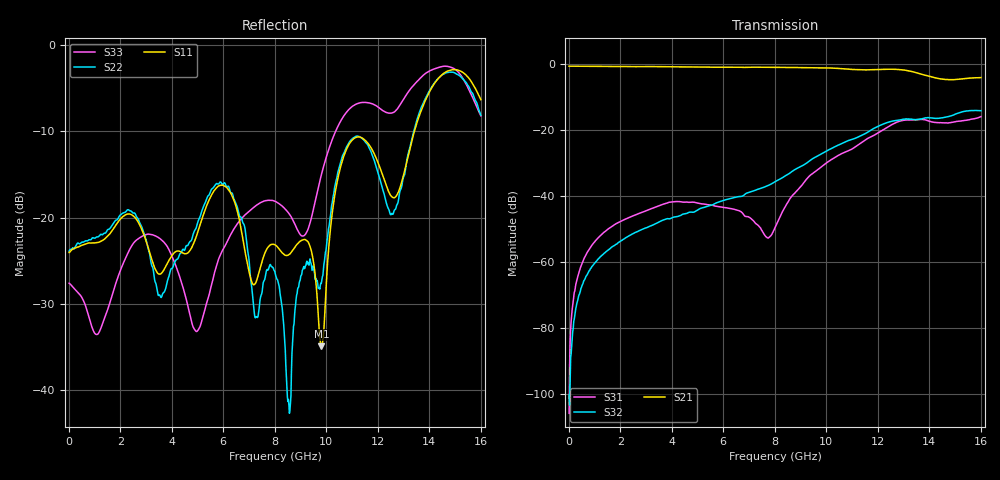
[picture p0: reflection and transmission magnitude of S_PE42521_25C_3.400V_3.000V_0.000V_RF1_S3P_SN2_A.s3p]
! Device ID: PE42521_Char_Units
! Serial: 2
! Insertion: A
! Temp: 25C
! VDD: 3.400
! Control_Hi: 3.000
! Control_Lo: 0.000
! Logic State: RF1
! ThroughPath: 2-1
! Port 1: RFC
! Port 2: RF1
! Port 3: RF2
! V1 = 3.00
! V2 = 0.00
! V3 = 0.00
! IDD: 1.364295e-04
! FILE NAME
! DATE 07-24-2013 19:14:31
! CORRECTED  DATA
#  Hz  S  RI  R  50
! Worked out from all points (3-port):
!   801 points, 10 MHz to 16.01 GHz, reference 50 ohm
!   strongest paths, dB at 10 MHz, 4.01 GHz, 8.01 GHz, 12.01 GHz, 16.01 GHz:
!     S21: -0.6, -0.8, -1.0, -1.6, -4.1
!     S32: -100.1, -46.5, -35.6, -18.8, -14.1
!     S31: -105.7, -41.7, -49.5, -20.9, -15.9
!   lowest |S11| = -34.9 dB at 9.81 GHz (marker M1), VSWR 1.04, Z = 48.5 - j1.02 ohm
!   |S11| at or under -10 dB: start of sweep to 13.43 GHz
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1e7  0.0628 -3.97e-05  0.9287 -0.00284  5.22e-06 2.55e-07
     0.9301 -0.00297  0.064 -0.000303  -3.27e-08 -1.37e-06
     1.71e-06 -4.88e-06  -3.36e-06 -9.25e-06  -0.0417 0.000256
6.5e8  0.0691 -0.0135  0.9117 -0.1498  -8.36e-05 0.00126
       0.9131 -0.1493  0.0721 -0.0132  -0.000164 0.000569
       -8.46e-05 0.00126  -0.000154 0.000567  -0.0306 0.00397
2.09e9  0.0892 0.0477  0.798 -0.4441  0.00125 0.00413
        0.7997 -0.4446  0.0944 0.0484  -9.73e-05 0.00219
        0.00125 0.00413  -0.000107 0.00219  -0.00571 0.0531
4.99e9  0.0701 -0.0402  0.3118 -0.8479  0.00671 0.00416
        0.3142 -0.8475  0.0725 -0.0565  0.000837 0.0061
        0.00673 0.00417  0.000821 0.00606  0.00249 -0.0219
8.01e9  -0.0577 -0.0389  -0.3495 -0.8197  -0.00105 0.00311
        -0.3457 -0.8202  -0.0383 0.0294  0.00327 0.0162
        -0.00107 0.00317  0.00317 0.0163  -0.1036 0.0688
8.55e9  -0.0193 -0.0579  -0.4594 -0.7601  -0.00482 0.00721
        -0.4547 -0.7617  -0.00336 -0.0075  0.00489 0.0214
        -0.00486 0.0071  0.00474 0.0214  -0.0973 0.041
9.81e9  -0.0146 -0.0105  -0.6819 -0.5544  -0.00687 0.0269
        -0.6806 -0.5572  0.0328 0.0257  0.0221 0.0377
        -0.00716 0.0268  0.0218 0.0378  0.00275 0.1765
1.091e10  -0.1165 0.2426  -0.7803 -0.2992  0.0092 0.0485
          -0.7793 -0.3027  -0.032 0.2735  0.0587 0.0397
          0.00877 0.0489  0.0582 0.0401  -0.0257 0.4258
1.403e10  0.3917 0.3727  -0.5373 0.3669  0.1207 -0.0631
          -0.5419 0.36  0.4312 0.3368  0.0746 -0.1347
          0.121 -0.0618  0.0753 -0.1337  0.6877 0.1661
1.601e10  0.3892 0.2834  -0.377 0.4986  0.0683 -0.143
          -0.3813 0.4953  0.2992 0.2534  -0.0842 -0.1796
          0.0704 -0.144  -0.0812 -0.1799  0.3514 0.1645
